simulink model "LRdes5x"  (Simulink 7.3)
settings: Solver=ode45  StartTime=0.0  StopTime=10.0  RelTol=1e-3
undefined symbols (not defined in the file or in its folder): Avl, Bvl, Cvl, Dvl

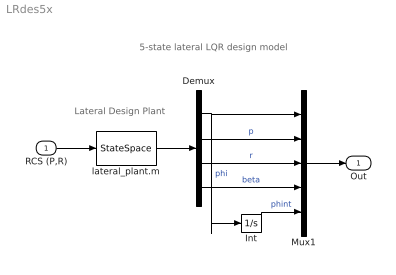
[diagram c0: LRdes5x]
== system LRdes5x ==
  note: 5-state lateral LQR design model
  note: Lateral Design Plant
  RCS (P,R) : Inport  OutDataType=sfix(16)  OutScaling=2^0
  Demux : Demux
  Int : Integrator
  Mux1 : Mux  Inputs=5
  lateral_plant.m : StateSpace  A=Avl  B=Bvl  C=Cvl  D=Dvl
  Out : Outport  OutDataType=sfix(16)  OutScaling=2^0
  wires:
  Mux1/1 -> Out/1
  RCS (P,R)/1 -> lateral_plant.m/1
  lateral_plant.m/1 -> Demux/1
  Demux/1 -> Mux1/1, Int/1  "phi"
  Demux/2 -> Mux1/2  "p"
  Demux/3 -> Mux1/3  "r"
  Demux/4 -> Mux1/4  "beta"
  Int/1 -> Mux1/5  "phint"
